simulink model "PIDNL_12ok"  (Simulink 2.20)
settings: Solver=VariableStepDiscrete  StartTime=0.0  StopTime=40.0  RelTol=1e-3  AbsTol=1e-6
undefined symbols (not defined in the file or in its folder): fnl, pidin
libraries: Puma x3, simulink x3

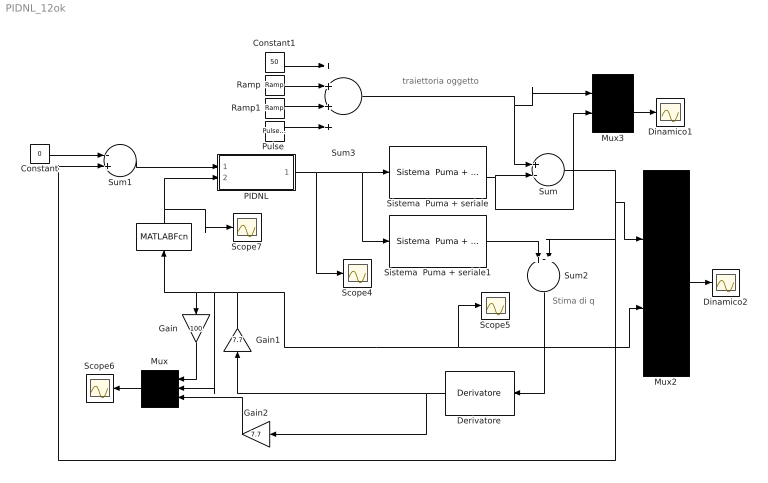
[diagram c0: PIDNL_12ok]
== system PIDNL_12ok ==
  note: Stima di q
  note: traiettoria oggetto
  " " : MATLABFcn  Orientation=up  MATLABFcn=fnl(u(1))  OutputWidth=-1
  Constant : Constant  Value=0
  Constant1 : Constant  Value=50
  Derivatore : Puma/Derivatore  Orientation=left  Td=0.13  T=0.033  N=10
  Dinamico1 : Scope
  Dinamico2 : Scope
  Gain : Gain  Orientation=down  Gain=100
  Gain1 : Gain  Orientation=up  Gain=7.7
  Gain2 : Gain  Orientation=left  Gain=7.7
  Mux : Mux  Orientation=left  Inputs=3
  Mux2 : Mux  Inputs=2
  Mux3 : Mux  Inputs=2
  PIDNL : Subsystem
  "Pulse " : simulink/Sources/Pulse Generator  period=30  duty=10  amplitude=-50  start=30
  Ramp : simulink/Sources/Ramp  slope=-50  start=10  X0=0
  Ramp1 : simulink/Sources/Ramp  slope=+50  start=25  X0=0
  Scope{4..7} (4 alike) : Scope
  Sistema  Puma + seriale : Puma/Sistema  Puma + seriale  Ts=.260
  Sistema  Puma + seriale1 : Puma/Sistema  Puma + seriale  Ts=.260
  Sum : Sum  Inputs=+-
  Sum1 : Sum  Inputs=-+
  Sum2 : Sum  Orientation=down  Inputs=++
  Sum3 : Sum  Inputs=++++
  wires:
  Sistema  Puma + seriale1/1 -> Sum2/1
  Mux2/1 -> Dinamico2/1
  Sistema  Puma + seriale/1 -> Sum/2, Mux3/2
  Sum2/1 -> Derivatore/1
  Mux/1 -> Scope6/1
  Derivatore/1 -> Gain2/1, Gain1/1
  Constant1/1 -> Sum3/1
  Sum1/1 -> PIDNL/1(In1)
  Constant/1 -> Sum1/1
  PIDNL/1(Out1) -> Sistema  Puma + seriale/1, Sistema  Puma + seriale1/1, Scope4/1
  Sum/1 -> Sum2/2, Sum1/2, Mux2/1
  Ramp/1 -> Sum3/2
  Ramp1/1 -> Sum3/3
  Gain2/1 -> Mux/3
  Gain/1 -> Mux/1
  Mux3/1 -> Dinamico1/1
  Sum3/1 -> Sum/1, Mux3/1
  Gain1/1 -> Gain/1, " "/1, Mux/2, Scope5/1, Mux2/2
  "Pulse "/1 -> Sum3/4
  " "/1 -> PIDNL/2(In2), Scope7/1

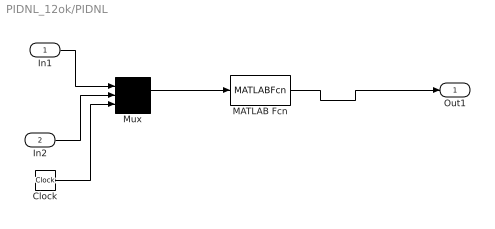
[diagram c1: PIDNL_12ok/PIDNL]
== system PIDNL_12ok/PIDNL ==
  In1 : Inport  Port=1  PortWidth=-1  SampleTime=-1
  In2 : Inport  Port=2  PortWidth=-1  SampleTime=-1
  Clock : Clock
  MATLAB Fcn : MATLABFcn  MATLABFcn=pidin(u(1),u(2),u(3))  OutputWidth=1
  Mux : Mux  Inputs=3
  Out1 : Outport  Port=1
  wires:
  MATLAB Fcn/1 -> Out1/1
  Mux/1 -> MATLAB Fcn/1
  In1/1 -> Mux/1
  In2/1 -> Mux/2
  Clock/1 -> Mux/3
